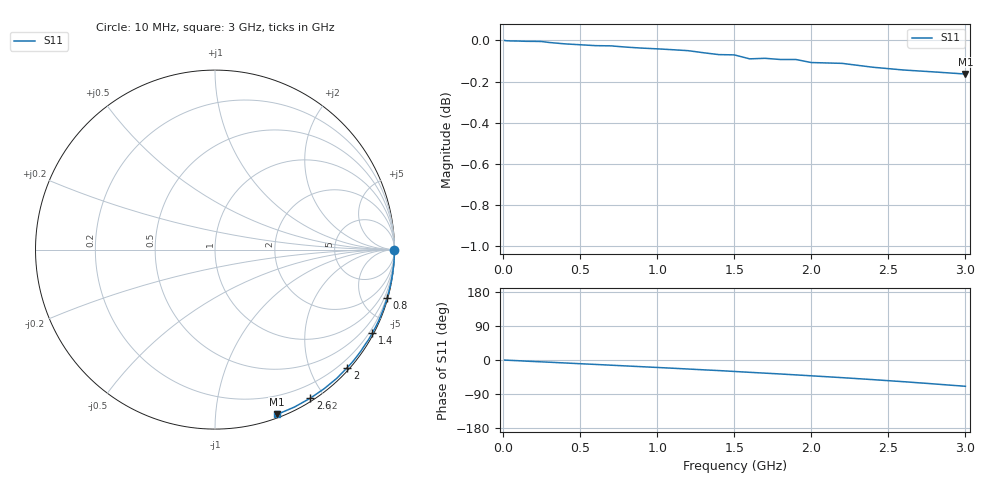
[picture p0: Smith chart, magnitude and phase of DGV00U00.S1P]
! SIEMENS Small Signal Semiconductors
! BAV70
! Silicon Switching Diode in SOT23
! VR = 0 V
! S-Parameters:  May  1995
# GHz  S  MA  R  50
!  f  S11
! GHz  MAG  ANG
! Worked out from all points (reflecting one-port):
!   30 points, 10 MHz to 3 GHz, reference 50 ohm
!   lowest |S11| = -0.2 dB at 3 GHz (marker M1), VSWR 106.35, Z = 1.45 - j72.2 ohm
!   phase of S11 starts at -0 deg and turns -69 deg over the sweep
!   S11 on the Smith chart (normalised r, x): 10 MHz: open; 800 MHz: 0.10, -7.25; 1.4 GHz: 0.07, -4.02; 2 GHz: 0.05, -2.62; 2.6 GHz: 0.04, -1.83; 3 GHz: 0.03, -1.44
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0.01  1 -0.2
0.05  0.9997 -1.0
0.1  0.9997 -1.9
0.15  0.9995 -3.0
0.2  0.9995 -4.0
0.25  0.9994 -4.9
0.3  0.9989 -5.8
0.4  0.9981 -7.8
0.5  0.9976 -9.8
0.6  0.9971 -11.7
0.7  0.997 -13.7
0.8  0.9963 -15.7
1  0.9953 -19.7
1.1  0.9948 -21.7
1.2  0.9943 -23.8
1.3  0.9931 -25.9
1.4  0.9921 -27.9
1.5  0.9919 -30.2
1.6  0.9898 -32.5
1.7  0.99 -34.7
1.8  0.9894 -36.9
1.9  0.9894 -39.3
2  0.9877 -41.7
2.2  0.9872 -46.6
2.4  0.9851 -51.8
2.6  0.9836 -57.3
2.8  0.9825 -63.2
3  0.9814 -69.4
